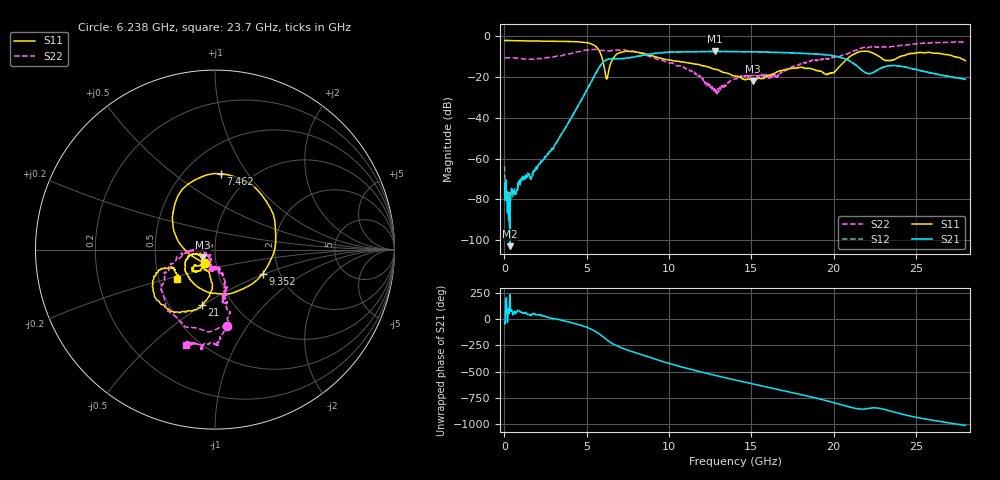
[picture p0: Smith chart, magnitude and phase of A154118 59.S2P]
!  2-Port S-parameters saved by WinCal
! VAR MeasName=S-Parameters (CALIBRATED_DATA) read from VNA (N5230A)
! VAR MeasDate=2015-9-10 14:39:39
! VAR NAME=A154118 59
! VAR FILENAME=A154118 59.S2P
! VAR DATE=2015-9-10 14:39:39
! VAR PHYS_PORTS=1,2
# Hz S DB R 50
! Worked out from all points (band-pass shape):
!   801 points, 10 MHz to 28 GHz, reference 50 ohm
!   highest |S21| = -7.52 dB at 12.78 GHz (marker M1); lowest = -102.9 dB at 324.9 MHz (marker M2)
!   |S21| within 3 dB of the highest: 7.668 GHz to 20.47 GHz (12.8 GHz wide, 91 % of centre)
!   lowest |S11| = -21.9 dB at 15.09 GHz (marker M3), VSWR 1.17, Z = 43.5 - j3.7 ohm
!   |S11| at or under -10 dB: 5.904 GHz to 6.686 GHz (782.2 MHz wide, 12.4 % of centre); 9.104 GHz to 21 GHz (11.9 GHz wide, 79.1 % of centre); 22.79 GHz to 24.03 GHz (1.247 GHz wide, 5.33 % of centre)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
!   |S22| runs from -28.4 to -2.8 dB; largest |S21 - S12| = 0.0079
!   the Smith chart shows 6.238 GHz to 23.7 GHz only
!   S11 on the Smith chart (normalised r, x): 6.238 GHz: 0.89, -0.14; 7.462 GHz: 0.73, +0.76; 9.352 GHz: 1.64, -0.48; 21 GHz: 0.72, -0.49; 23.7 GHz: 0.62, -0.22
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1e7  -2.15 179.7  -72.00 -30.4  -63.63 -74.6  -10.72 179.8
3.248875e8  -2.19 175.2  -102.86 -126.1  -88.46 -42.8  -10.61 166.2
2.66905e9  -2.46 143.8  -57.61 13.9  -57.75 13.4  -10.53 71.6
4.698325e9  -3.02 98.2  -31.00 -62.5  -30.96 -62.9  -7.34 -22.6
5.677975e9  -6.18 36.5  -16.34 -132.1  -16.33 -132.2  -6.72 -65.1
6.237775e9  -20.56 -125.1  -11.50 160.0  -11.48 159.9  -7.34 -80.8
6.7276e9  -9.60 133.2  -11.14 112.5  -11.15 112.5  -6.76 -94.1
7.462338e9  -7.46 85.8  -10.73 65.6  -10.75 65.7  -7.15 -117.1
9.351662e9  -10.51 -26.8  -8.32 -32.2  -8.28 -32.1  -11.46 -160.6
1.085612e10  -12.76 -112.4  -7.69 -100.5  -7.64 -101.1  -15.17 -170.8
1.278044e10  -16.23 -164.6  -7.52 -175.6  -7.48 -176.2  -25.01 -137.8
1.4005e10  -19.60 -168.0  -7.64 139.7  -7.61 139.2  -21.02 -105.3
1.508961e10  -21.91 -148.2  -7.66 101.9  -7.65 101.3  -18.22 -96.6
1.715388e10  -16.16 -128.7  -8.13 30.0  -8.07 29.6  -16.69 -71.2
1.869332e10  -16.01 -140.8  -8.71 -24.2  -8.75 -25.0  -11.65 -76.9
1.991789e10  -17.87 -109.6  -9.58 -72.4  -9.61 -73.3  -10.32 -80.2
2.10025e10  -10.01 -103.1  -12.33 -120.0  -12.31 -121.0  -7.92 -79.6
2.21221e10  -7.59 -144.7  -18.41 -131.8  -18.39 -133.0  -5.52 -93.8
2.334666e10  -12.03 -149.0  -14.49 -152.7  -14.52 -153.3  -5.43 -105.8
2.369654e10  -11.47 -142.6  -14.42 -167.8  -14.42 -168.2  -5.07 -107.1
2.57608e10  -7.93 -167.0  -17.77 122.4  -17.83 121.3  -3.47 -122.9
2.8e10  -12.10 158.5  -21.12 66.0  -21.12 65.9  -2.76 -140.5
